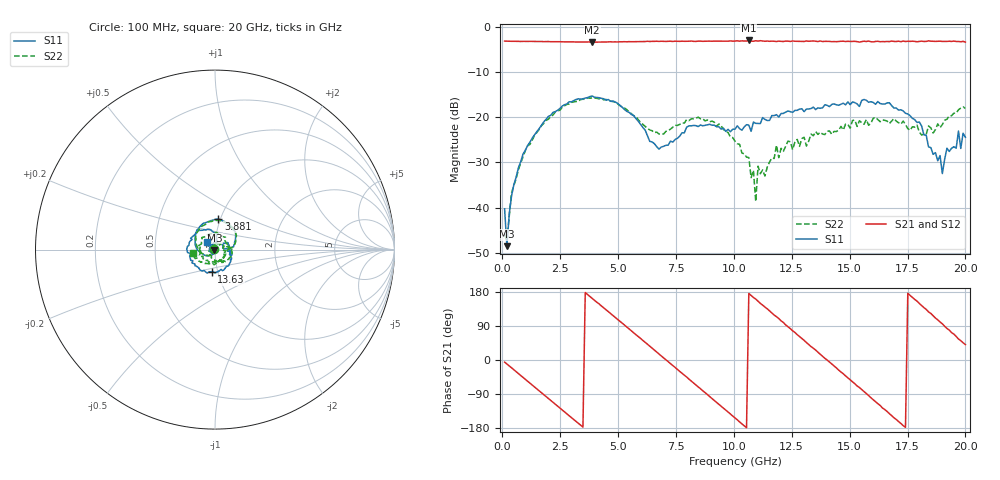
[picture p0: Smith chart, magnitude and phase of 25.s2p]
!Agilent Technologies,N5230C,MY49001569,A.09.33.09
!Agilent N5230C: A.09.33.09
!Date: Monday, July 27, 2015 10:28:17
!Correction: S11(Full 2 Port(1,2))
!S21(Full 2 Port(1,2))
!S12(Full 2 Port(1,2))
!S22(Full 2 Port(1,2))
!S2P File: Measurements: S11, S21, S12, S22:
# Hz S  dB  R 50
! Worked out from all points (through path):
!   201 points, 100 MHz to 20 GHz, reference 50 ohm
!   highest |S21| = -2.96 dB at 10.65 GHz (marker M1); lowest = -3.3 dB at 3.881 GHz (marker M2)
!   group delay of S21, straight-line fit = 144 ps
!   lowest |S11| = -48.6 dB at 199.5 MHz (marker M3), VSWR 1.01, Z = 49.7 - j0.229 ohm
!   |S11| at or under -10 dB: start of sweep to end of sweep
!   |S22| runs from -47.5 to -15.7 dB; largest |S21 - S12| = 0.03
!   S11 on the Smith chart (normalised r, x): 100 MHz: 0.98, +0.00; 3.881 GHz: 0.98, +0.35; 13.63 GHz: 0.93, -0.24; 20 GHz: 0.91, +0.08
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1e8  -40.30 173.9  -3.10 -5.6  -3.11 -5.0  -45.90 149.1
1.995e8  -48.56 -141.8  -3.12 -10.5  -3.10 -10.6  -47.52 -88.0
8.96e8  -28.14 -123.9  -3.17 -45.9  -3.16 -46.1  -28.74 -123.5
2.09e9  -19.57 173.4  -3.24 -106.8  -3.24 -107.1  -19.84 170.4
3.483e9  -15.89 102.6  -3.30 -177.0  -3.31 -177.6  -15.99 101.7
3.881e9  -15.27 83.6  -3.35 162.5  -3.35 162.4  -15.67 82.3
5.274e9  -18.25 23.9  -3.23 92.4  -3.27 91.9  -17.93 24.0
6.7665e9  -27.06 11.9  -3.17 16.1  -3.13 15.9  -23.71 8.6
8.657e9  -21.88 16.2  -3.15 -81.1  -3.12 -81.7  -20.29 -25.1
1.005e10  -22.63 -2.8  -3.08 -153.0  -3.08 -153.5  -25.31 -98.1
1.0647e10  -21.74 -8.4  -2.96 175.5  -3.07 175.3  -28.92 -168.5
1.09455e10  -21.34 -10.8  -3.03 160.8  -3.04 159.5  -38.64 179.6
1.1045e10  -21.36 -7.2  -3.11 155.2  -3.08 154.5  -30.82 153.3
1.2239e10  -18.85 -46.4  -3.10 92.6  -3.10 92.6  -26.39 33.7
1.3433e10  -17.74 -90.2  -3.07 31.1  -3.17 30.2  -24.09 -43.6
1.3632e10  -17.90 -98.5  -3.21 20.5  -3.19 19.7  -23.79 -49.5
1.5423e10  -17.59 -169.4  -3.33 -72.7  -3.17 -74.7  -20.76 178.9
1.67165e10  -16.77 132.8  -3.21 -141.6  -3.21 -141.8  -21.38 97.9
1.77115e10  -20.24 95.2  -3.12 165.1  -3.12 164.4  -22.09 16.8
1.87065e10  -27.83 94.3  -3.17 110.8  -3.13 110.4  -22.72 -81.2
1.9005e10  -32.47 107.7  -3.18 95.5  -3.10 93.6  -21.60 -106.2
2e10  -24.43 136.8  -3.33 40.6  -3.23 39.6  -18.04 -171.0
